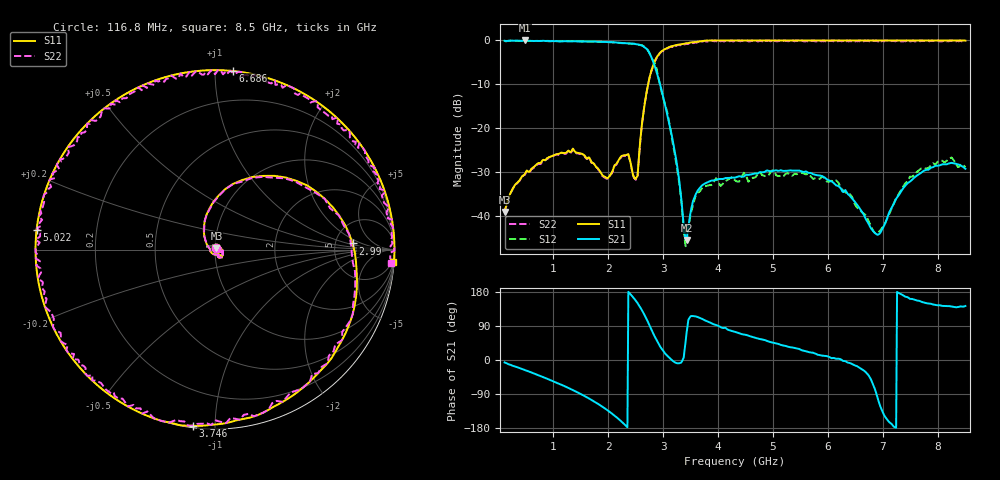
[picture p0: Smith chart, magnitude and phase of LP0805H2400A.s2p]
!	AVX	THIN	FILM	OPERATION
!	LP0805	High	Performance	Low	Pass	Filter	P/N	LP0805H2400ASTR
!	November	"13,"	2016
!Instrument:	"HEWLETT PACKARD,8720ES,US39172150,7.62 "
#	MHz	S	dB	R	50
!	Frq	S11(dB)	S11(deg)	S21(dB)	S21(deg)	S12(dB)	S12(deg)	S22(dB)	S22(deg)
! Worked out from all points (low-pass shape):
!   500 points, 116.8 MHz to 8.5 GHz, reference 50 ohm
!   highest |S21| = 0.00 dB at 486.4 MHz (marker M1); lowest = -45.4 dB at 3.426 GHz (marker M2)
!   |S21| within 3 dB of the highest: start of sweep to 2.757 GHz
!   lowest |S11| = -39.0 dB at 116.8 MHz (marker M3), VSWR 1.02, Z = 50.8 + j0.781 ohm
!   |S11| at or under -10 dB: start of sweep to 2.727 GHz
!   |S22| runs from -39.2 to 0.0 dB; largest |S21 - S12| = 0.085
!   S11 on the Smith chart (normalised r, x): 116.8 MHz: 1.02, +0.02; 2.99 GHz: 7.39, +1.24; 3.746 GHz: 0.01, -0.88; 5.022 GHz: -0.00, +0.05; 6.686 GHz: 0.00, +1.10; 8.5 GHz: 2, -28
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116.8  -38.97 43.0  -0.07 -6.4  -0.12 -6.6  -39.17 43.0
486.4  -30.35 12.9  0.00 -27.0  -0.01 -26.4  -30.55 12.8
1528  -25.79 -62.2  -0.21 -91.6  -0.23 -91.7  -25.99 -62.2
1964.8  -31.18 -44.1  -0.36 -130.1  -0.35 -130.3  -31.38 -44.3
2384.8  -26.65 -41.8  -0.68 177.3  -0.72 176.6  -26.75 -41.8
2519.2  -31.11 -160.1  -0.86 153.4  -0.84 152.6  -31.11 -160.3
2687.2  -12.71 97.7  -1.79 111.6  -1.66 111.2  -12.91 97.6
2804.8  -6.19 56.8  -4.34 74.8  -4.26 76.6  -6.29 56.7
2922.4  -3.14 20.0  -8.92 41.8  -8.77 35.7  -3.34 19.9
2989.6  -2.30 2.6  -12.19 26.9  -12.56 23.5  -2.40 2.4
3224.8  -1.11 -40.5  -26.12 -6.9  -26.86 -13.2  -1.21 -40.6
3426.4  -0.65 -65.9  -45.36 70.2  -46.63 74.5  -0.65 -66.0
3577.6  -0.38 -81.6  -35.46 115.5  -35.86 117.8  -0.38 -81.8
3745.6  -0.09 -97.3  -32.63 105.7  -33.23 106.5  -0.09 -97.4
4316.8  0.00 -140.9  -31.14 74.0  -31.86 71.6  -0.20 -141.1
5022.4  0.00 173.8  -29.60 44.8  -29.71 42.0  -0.10 173.6
5711.2  0.00 135.6  -30.28 19.4  -31.24 26.6  0.00 135.4
6685.6  0.00 84.3  -40.53 -31.9  -39.73 -31.0  -0.10 84.1
6904  0.00 73.2  -44.20 -101.2  -43.73 -94.5  -0.20 73.2
7105.6  0.00 63.1  -39.36 -162.5  -39.71 -155.2  -0.20 62.9
7676.8  0.00 35.5  -30.24 155.1  -29.30 158.8  -0.20 35.5
8500  -0.04 -4.1  -29.17 142.5  -28.82 144.1  -0.14 -4.2
